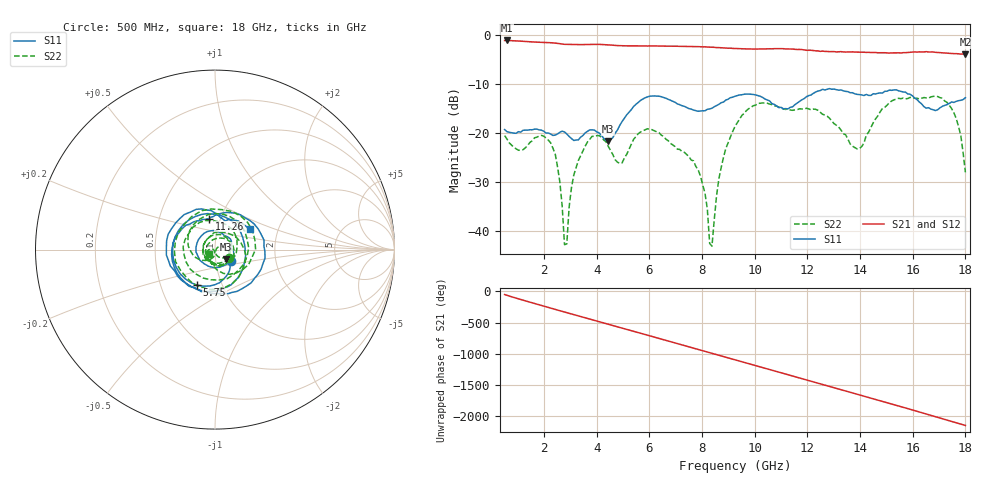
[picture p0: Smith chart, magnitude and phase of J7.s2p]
!Agilent Technologies,N5230A,MY45001360,A.07.50.67
!Agilent N5230A: A.07.50.67
!Date: Tuesday, April 16, 2024 16:02:00
!Correction: S11(Full 2 Port(1,2))
!S21(Full 2 Port(1,2))
!S12(Full 2 Port(1,2))
!S22(Full 2 Port(1,2))
!S2P File: Measurements: S11, S21, S12, S22:
# Hz S  dB  R 50
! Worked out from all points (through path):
!   201 points, 500 MHz to 18 GHz, reference 50 ohm
!   highest |S21| = -1.19 dB at 587.5 MHz (marker M1); lowest = -4.0 dB at 18 GHz (marker M2)
!   group delay of S21, straight-line fit = 331 ps
!   lowest |S11| = -21.7 dB at 4.438 GHz (marker M3), VSWR 1.18, Z = 56.3 - j6.09 ohm
!   |S11| at or under -10 dB: start of sweep to end of sweep
!   |S22| runs from -43.0 to -12.5 dB; largest |S21 - S12| = 0.0077
!   S11 on the Smith chart (normalised r, x): 500 MHz: 1.18, -0.15; 5.75 GHz: 0.76, -0.32; 11.26 GHz: 0.88, +0.32; 18 GHz: 1.43, +0.36
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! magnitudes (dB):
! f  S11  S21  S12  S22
! 500 MHz  -19.3  -1.2  -1.2  -20.5
! 587.5 MHz  -19.7  -1.2  -1.2  -21.2
! 2.25 GHz  -20.2  -1.7  -1.6  -22.0
! 2.6 GHz  -19.9  -1.8  -1.8  -30.0
! 2.775 GHz  -19.8  -2.0  -2.0  -42.7
! 3.125 GHz  -21.5  -2.0  -2.0  -28.6
! 3.475 GHz  -20.5  -2.0  -2.0  -23.6
! 4.438 GHz  -21.7  -2.1  -2.1  -22.7
! 4.963 GHz  -17.7  -2.3  -2.3  -26.1
! 5.75 GHz  -13.1  -2.3  -2.3  -19.6
! 6.362 GHz  -12.5  -2.3  -2.3  -19.9
! 7.85 GHz  -15.6  -2.4  -2.5  -27.5
! 8.375 GHz  -15.0  -2.5  -2.6  -43.0
! 8.637 GHz  -14.2  -2.6  -2.6  -29.3
! 9.25 GHz  -12.5  -2.8  -2.8  -18.7
! 11.26 GHz  -15.1  -2.9  -2.9  -15.1
! 12.22 GHz  -11.9  -3.2  -3.2  -15.2
! 13.89 GHz  -12.2  -3.6  -3.5  -23.3
! 15.11 GHz  -11.3  -3.8  -3.7  -13.8
! 17.3 GHz  -14.2  -3.8  -3.8  -13.8
! 17.74 GHz  -13.4  -3.9  -3.9  -18.7
! 18 GHz  -12.8  -4.0  -4.0  -28.0
